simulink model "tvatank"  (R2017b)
settings: Solver=VariableStepAuto  StartTime=0.0  StopTime=100  RelTol=1e-3
libraries: simulink x1

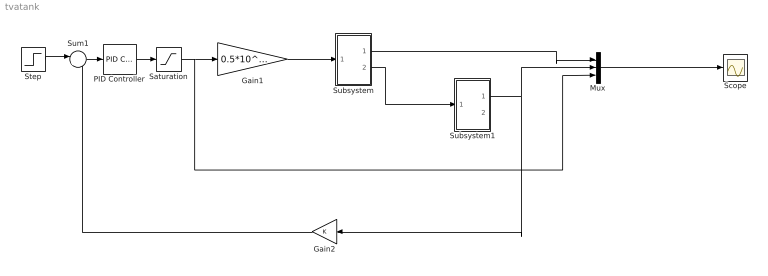
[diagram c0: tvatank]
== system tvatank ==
  Gain1 : Gain  Gain=0.5*10^(-5)
  Gain2 : Gain
  Mux : Mux  Inputs=3
  PID Controller : simulink/Continuous/PID Controller  Controller=PI  TimeDomain=Continuous-time  SampleTime=-1  IntegratorMethod=Forward Euler  FilterMethod=Forward Euler  Form=Parallel  UseFilter=on  ControllerParametersSource=internal  P=0.1  I=1.2  D=0  N=100  InitialConditionSource=internal  InitialConditionForIntegrator=0  InitialConditionForFilter=0  ExternalReset=none  LimitOutput=off  UpperSaturationLimit=inf  LowerSaturationLimit=-inf  LinearizeAsGain=on  AntiWindupMode=none  Kb=1  TrackingMode=off  Kt=1  PParamMin=[]  PParamMax=[]  IParamMin=[]  IParamMax=[]  DParamMin=[]  DParamMax=[]  NParamMin=[]  NParamMax=[]  KbParamMin=[]  KbParamMax=[]  KtParamMin=[]  KtParamMax=[]  POutMin=[]  POutMax=[]  IOutMin=[]  IOutMax=[]  DOutMin=[]  DOutMax=[]  NOutMin=[]  NOutMax=[]  KbOutMin=[]  KbOutMax=[]  KtOutMin=[]  KtOutMax=[]  IntegratorOutMin=[]  IntegratorOutMax=[]  FilterOutMin=[]  FilterOutMax=[]  SumOutMin=[]  SumOutMax=[]  SumI1OutMin=[]  SumI1OutMax=[]  SumI2OutMin=[]  SumI2OutMax=[]  SumI3OutMin=[]  SumI3OutMax=[]  SumDOutMin=[]  SumDOutMax=[]  SaturationOutMin=[]  SaturationOutMax=[]  IntegratorContinuousStateAttributes=''  IntegratorStateMustResolveToSignalObject=off  IntegratorRTWStateStorageClass=Auto  FilterContinuousStateAttributes=''  FilterStateMustResolveToSignalObject=off  FilterRTWStateStorageClass=Auto  DifferentiatorICPrevScaledInput=0  DifferentiatorOutMin=[]  DifferentiatorOutMax=[]  InitialConditionSetting=State (most efficient)  FilterDiffOutCoefMin=[]  FilterDiffOutCoefMax=[]  SumDenOutMin=[]  SumDenOutMax=[]  SumNumOutMin=[]  SumNumOutMax=[]  ReciprocalOutMin=[]  ReciprocalOutMax=[]  DivideOutMin=[]  DivideOutMax=[]  TunerSelectOption=Transfer Function Based (PID Tuner App)
  Saturation : Saturate  UpperLimit=5  LowerLimit=0
  Scope : Scope
  Step : Step  Before=1  SampleTime=0
  Subsystem : Subsystem
  Subsystem1 : Subsystem
  Sum1 : Sum  Inputs=|+-
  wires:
  PID Controller/1 -> Saturation/1
  Step/1 -> Sum1/1
  Sum1/1 -> PID Controller/1
  Gain2/1 -> Sum1/2
  Mux/1 -> Scope/1
  Subsystem/1(Out1) -> Mux/1
  Gain1/1 -> Subsystem/1(In1)
  Subsystem/2(Out2) -> Subsystem1/1(In1)
  Subsystem1/1(Out1) -> Gain2/1, Mux/2
  Saturation/1 -> Mux/3, Gain1/1

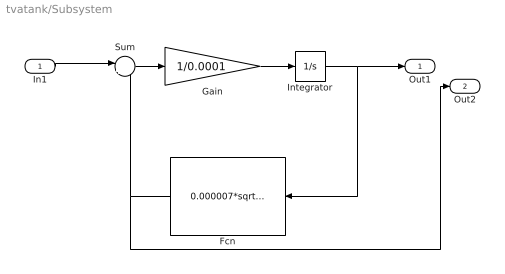
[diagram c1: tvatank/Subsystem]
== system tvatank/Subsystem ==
  In1 : Inport
  Fcn : Fcn  Expr=0.000007*sqrt(2*9.81*u)
  Gain : Gain  Gain=1/0.0001
  Integrator : Integrator
  Sum : Sum  Inputs=|+-
  Out1 : Outport
  Out2 : Outport  Port=2
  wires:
  Integrator/1 -> Out1/1, Fcn/1
  Sum/1 -> Gain/1
  Gain/1 -> Integrator/1
  In1/1 -> Sum/1
  Fcn/1 -> Out2/1, Sum/2

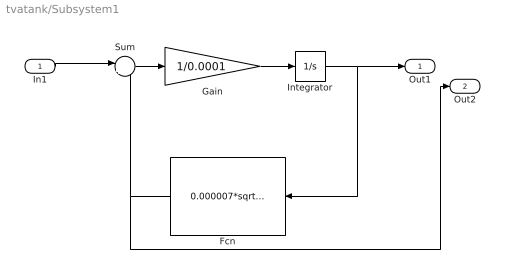
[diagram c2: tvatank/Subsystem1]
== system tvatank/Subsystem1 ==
  In1 : Inport
  Fcn : Fcn  Expr=0.000007*sqrt(2*9.81*u)
  Gain : Gain  Gain=1/0.0001
  Integrator : Integrator
  Sum : Sum  Inputs=|+-
  Out1 : Outport
  Out2 : Outport  Port=2
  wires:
  Integrator/1 -> Out1/1, Fcn/1
  Sum/1 -> Gain/1
  Gain/1 -> Integrator/1
  In1/1 -> Sum/1
  Fcn/1 -> Out2/1, Sum/2
